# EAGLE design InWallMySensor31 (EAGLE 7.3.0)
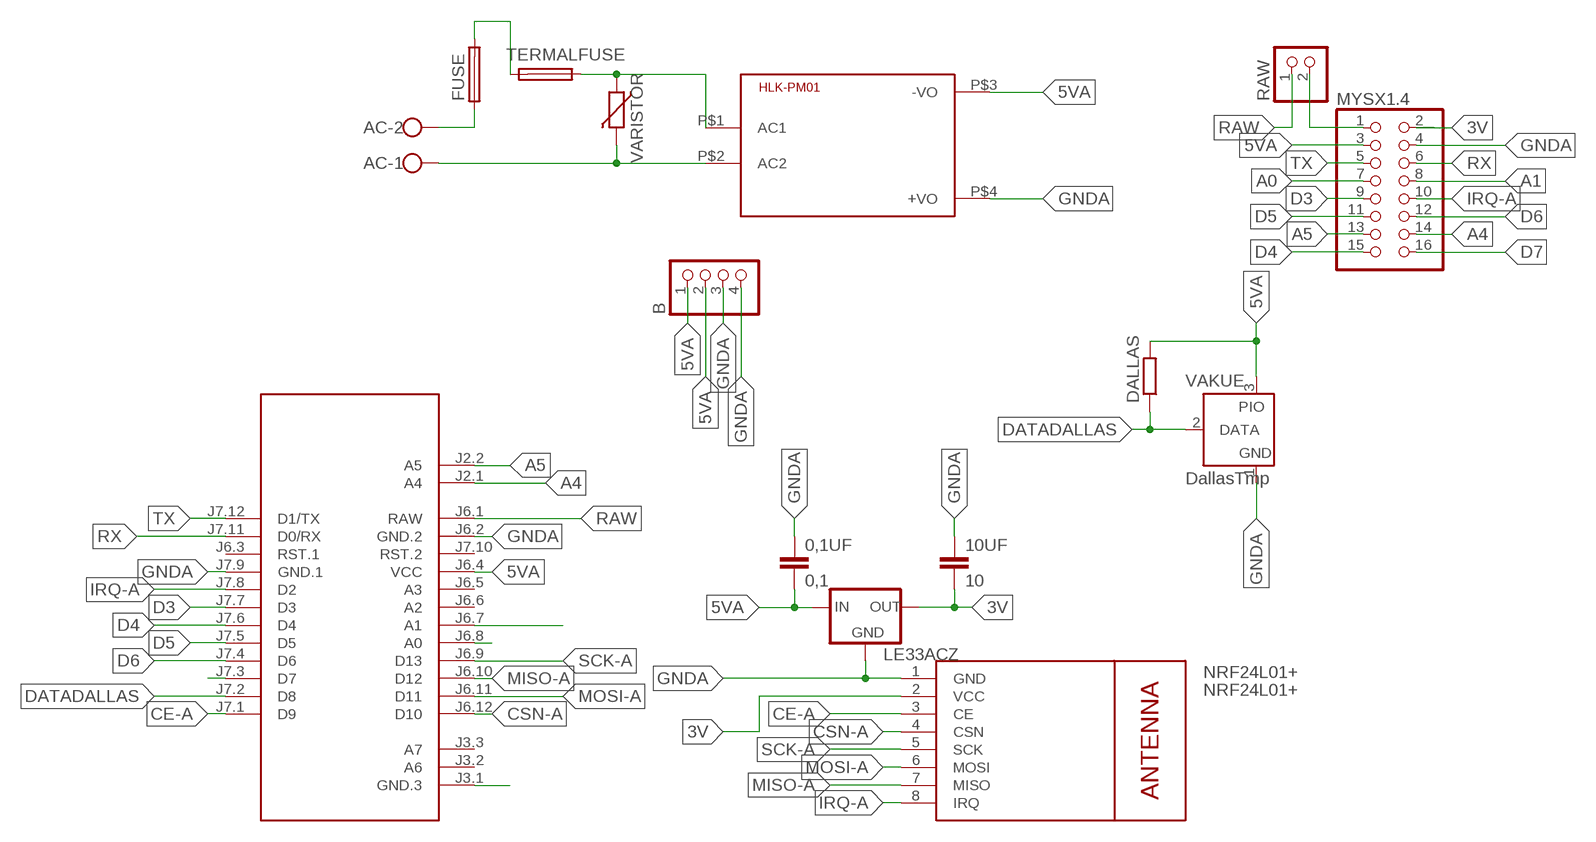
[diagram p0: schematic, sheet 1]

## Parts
0,1UF  0,1  C5/2.5  [C5B2.5]
10UF  10  C5/2.5  [C5B2.5]
AC  W237-102  [W237-102]
B  PINHD-1X04_2.54-S  [1X04-S]
DALLAS  R-EU_0204/5  [0204/5]
FUSE  FUSETE5  [TE5]
HLK-PM01  HKLPM01  [HKLPM01]
LE33ACZ  78LXX  [78LXX]
M1  ARDUINO-PRO-MINI-3.3V#NP  [ARDUINO-PRO-MINI#NP]
MYSX1.4  PINHD-2X08_2.54  [2X08]
NRF24L01+  NRF24L01+  WIRELESS-NRF24L01  [WIRELESS-NRF24L01]
RAW  PINHD-1X02_2.54-S  [1X02-S]
TERMALFUSE  FUSETE5  [TE5]
VAKUE  DallasTmp  DS2405  [TO92-]
VARISTOR  VARISTOR-7,5  [R-7,5]

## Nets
3V: 10UF.2 LE33ACZ.OUT MYSX1.4.2 NRF24L01+.2(VCC)
5VA: 0,1UF.2 B.1 B.2 DALLAS.2 HLK-PM01.P$3(-VO) LE33ACZ.IN M1.J6.4(VCC) MYSX1.4.3 VAKUE.3(PIO)
A0: M1.J6.8(A0) MYSX1.4.7
A1: M1.J6.7(A1) MYSX1.4.8
A4: M1.J2.1(A4) MYSX1.4.14
A5: M1.J2.2(A5) MYSX1.4.13
ACGND: AC.1 HLK-PM01.P$2(AC2) VARISTOR.2
CE-A: M1.J7.1(D9) NRF24L01+.3(CE)
CSN-A: M1.J6.12(D10) NRF24L01+.4(CSN)
D3: M1.J7.7(D3) MYSX1.4.9
D4: M1.J7.6(D4) MYSX1.4.15
D5: M1.J7.5(D5) MYSX1.4.11
D6: M1.J7.4(D6) MYSX1.4.12
D7: M1.J7.3(D7) MYSX1.4.16
DATADALLAS: DALLAS.1 M1.J7.2(D8) VAKUE.2(DATA)
GNDA: 0,1UF.1 10UF.1 B.3 B.4 HLK-PM01.P$4(+VO) LE33ACZ.GND M1.J6.2(GND.2) M1.J7.9(GND.1) MYSX1.4.4 NRF24L01+.1(GND) VAKUE.1(GND)
IRQ-A: M1.J7.8(D2) MYSX1.4.10 NRF24L01+.8(IRQ)
MISO-A: M1.J6.10(D12) NRF24L01+.7(MISO)
MOSI-A: M1.J6.11(D11) NRF24L01+.6(MOSI)
N$1: FUSE.2 TERMALFUSE.2
N$4: AC.2 FUSE.1
N$5: M1.J3.1(GND.3)
N$6: MYSX1.4.1 RAW.2
N$7: HLK-PM01.P$1(AC1) TERMALFUSE.1 VARISTOR.1
RAW: M1.J6.1(RAW) RAW.1
RX: M1.J7.11(D0/RX) MYSX1.4.6
SCK-A: M1.J6.9(D13) NRF24L01+.5(SCK)
TX: M1.J7.12(D1/TX) MYSX1.4.5
Unconnected: M1.J3.2(A6) M1.J3.3(A7) M1.J6.3(RST.1) M1.J6.5(A3) M1.J6.6(A2) M1.J7.10(RST.2)

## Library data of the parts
0,1UF 10UF = capacitor-wima:C: CAPACITOR
AC = con-wago-500:W237-102: WAGO SCREW CLAMP; MPN: 237-102; OC_FARNELL: unknown; OC_NEWARK: 70K9898
B = pinhead-2:PINHD-1X04: PIN HEADER
DALLAS = resistor:R-EU_: RESISTOR, European symbol
FUSE TERMALFUSE = fuse:FUSE: Fuse; OC_FARNELL: unknown; OC_NEWARK: unknown
HLK-PM01 = HKLPM01:HKLPM01
LE33ACZ = v-reg:78LXX: VOLTAGE REGULATOR
M1 = diy-modules:ARDUINO-PRO-MINI-*#NP: Arduino Pro Mini without programming pads
MYSX1.4 = pinhead-2:PINHD-2X08: PIN HEADER
NRF24L01+ = diy-modules:WIRELESS-NRF24L01: 2.4 GHz Wireless Module based on NRF24L01 chip
RAW = pinhead-2:PINHD-1X02: PIN HEADER
VAKUE = maxim:DS2405: Addressable Switch DALLAS Semiconductor; MF: DALLAS SEMICONDUCTOR; MPN: DS2405; OC_FARNELL: 1188025; OC_NEWARK: 06F4645
VARISTOR = varistor:VARISTOR: VARISTOR

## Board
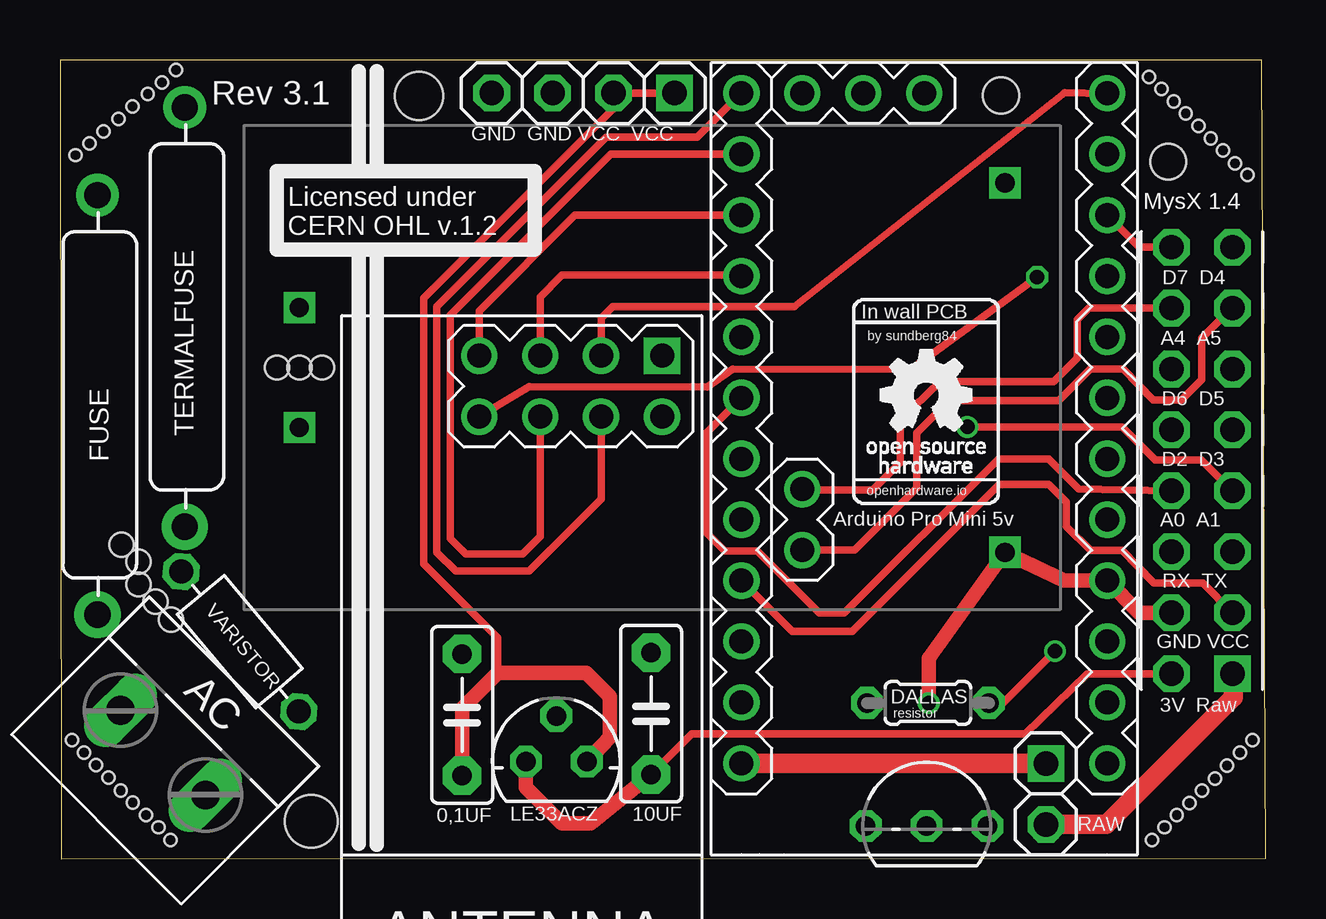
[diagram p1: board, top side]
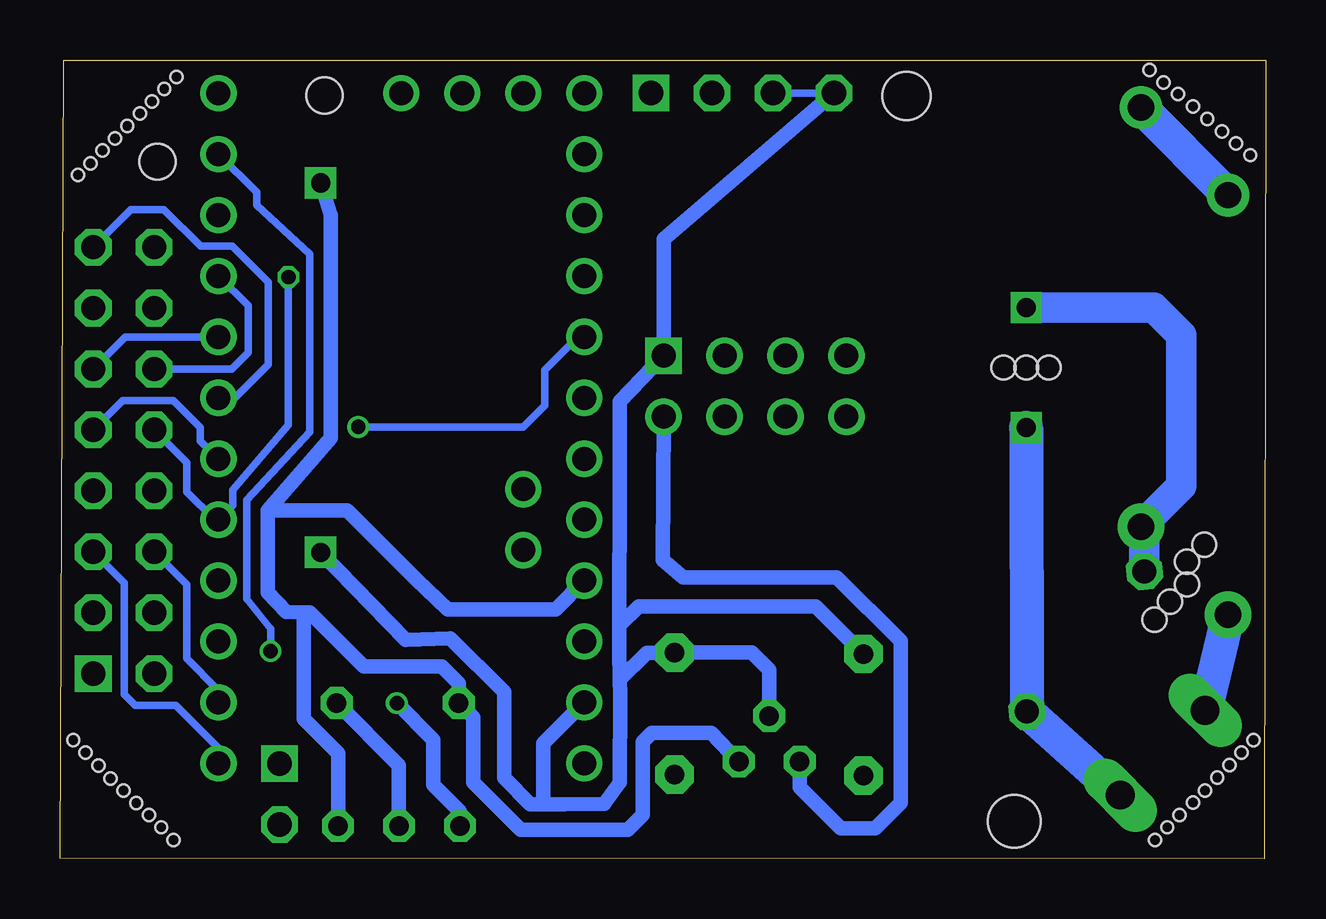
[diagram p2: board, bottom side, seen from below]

Size 50.23 x 33.31 mm. Coordinates in mm from the lower left corner, seen from the top.
Outline: 0.05,0 50.23,0.03 50.08,33.31 0,33.31 0.05,0
Copper layers (1*16): Top 0.035mm / dielectric 1.5mm / Bottom 0.035mm
Design rules "ITead_rule": minimum track width 6mil, minimum drill 12mil, track to track 6mil, track to pad 6mil, pad to pad 6mil, via to via 6mil, smd to smd 0mil, copper to edge 10mil, drill to drill 10mil, minimum pad ring 10mil, minimum via ring 6mil, stop-mask expansion 2mil, vias tented up to drill 100mil, thermal gap 10mil
Holes 2 mm at 14.96,31.81
Holes 2.2 mm at 10.47,1.56
Holes 1.5 mm at 39.2,31.83 46.18,29.07
Holes 0.5 mm at 45.38,32.61 46.41,31.58 47.43,30.56 48.46,29.53 49.48,28.51 45.51,0.78 46.53,1.83 47.58,2.86 48.63,3.88 49.68,4.96 4.61,0.78 3.58,1.83 2.53,2.86 1.51,3.91 0.51,4.96 4.83,32.88 3.66,31.88 2.43,30.86 1.23,29.83 4.1,1.32 3.03,2.36 2.02,3.4 1,4.44 0.64,29.34 1.81,30.33 3.03,31.37 4.25,32.36 45.89,32.1 46.91,31.08 47.95,30.04 48.96,29 46.01,1.32 47.06,2.33 48.12,3.35 49.16,4.44
Holes 1 mm at 3.27,12.38 3.27,11.44 3.98,10.73 9.97,20.48 9.03,20.48 10.91,20.48 2.56,13.09 4.63,9.98

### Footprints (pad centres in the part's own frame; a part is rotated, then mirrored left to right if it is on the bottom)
C5B2.5 = drill 0.813 pad 1.6 octagon: 1 -2.54,0; 2 2.54,0
W237-102 = drill 1.194 long: 1 -2.5,-1.27; 2 2.5,-1.27
1X04-S = drill 1.016 square: 1 -3.81,0 | drill 1.016 octagon: 2 -1.27,0; 3 1.27,0; 4 3.81,0
0204/5 = drill 0.813 octagon: 1 -2.54,0; 2 2.54,0
TE5 = drill 1.1 pad 1.93: 1 -5.632,0 | drill 1.1 pad 1.778: 2 11.852,0
HKLPM01 = drill 0.8 square: P$1 -14.7,2.5; P$2 -14.7,-2.5; P$3 14.7,7.7; P$4 14.7,-7.7
78LXX = drill 0.813 octagon: GND 0,1.905; IN 1.27,0; OUT -1.27,0
ARDUINO-PRO-MINI#NP = drill 1: J2.1 -1.27,5.08; J2.2 -3.81,5.08; J3.1 15.24,0; J3.2 15.24,2.54; J3.3 15.24,5.08; J6.1 -12.7,7.62; J6.2 -10.16,7.62; J6.3 -7.62,7.62; J6.4 -5.08,7.62; J6.5 -2.54,7.62; J6.6 0,7.62; J6.7 2.54,7.62; J6.8 5.08,7.62; J6.9 7.62,7.62; J6.10 10.16,7.62; J6.11 12.7,7.62; J6.12 15.24,7.62; J7.1 15.24,-7.62; J7.2 12.7,-7.62; J7.3 10.16,-7.62; J7.4 7.62,-7.62; J7.5 5.08,-7.62; J7.6 2.54,-7.62; J7.7 0,-7.62; J7.8 -2.54,-7.62; J7.9 -5.08,-7.62; J7.10 -7.62,-7.62; J7.11 -10.16,-7.62; J7.12 -12.7,-7.62
2X08 = drill 1.016 square: 1 -8.89,-1.27 | drill 1.016 octagon: 2 -8.89,1.27; 3 -6.35,-1.27; 4 -6.35,1.27; 5 -3.81,-1.27; 6 -3.81,1.27; 7 -1.27,-1.27; 8 -1.27,1.27; 9 1.27,-1.27; 10 1.27,1.27; 11 3.81,-1.27; 12 3.81,1.27; 13 6.35,-1.27; 14 6.35,1.27; 15 8.89,-1.27; 16 8.89,1.27
WIRELESS-NRF24L01 = drill 1 square: 1 -12.7,6.35 | drill 1: 2 -10.16,6.35; 3 -12.7,3.81; 4 -10.16,3.81; 5 -12.7,1.27; 6 -10.16,1.27; 7 -12.7,-1.27; 8 -10.16,-1.27
1X02-S = drill 1.016 square: 1 -1.27,0 | drill 1.016 octagon: 2 1.27,0
TO92- = drill 0.813 octagon: 1 -2.54,0; 2 0,0; 3 2.54,0
R-7,5 = drill 1 octagon: 1 -3.81,0; 2 3.81,0

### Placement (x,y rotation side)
0,1UF  16.76,6.01 270 top
10UF  24.63,6.06 270 top
AC  3.39,3.53 135 top
B  21.8,31.93 180 top
DALLAS  36.16,6.5 180 top
FUSE  1.56,15.82 90 top
HLK-PM01  24.67,20.48 0 top
LE33ACZ  20.68,4.06 0 top
M1  36.01,16.68 90 top
MYSX1.4  47.58,16.61 90 top
NRF24L01+  18.73,8.28 270 top
RAW  41.08,2.71 270 top
TERMALFUSE  5.2,19.48 90 top
VAKUE  36.11,1.37 0 top
VARISTOR  7.5,9.06 310 top

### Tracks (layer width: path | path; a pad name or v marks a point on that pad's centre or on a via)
3V
  Top 0.305: MYSX1.4.2 42.8,7.72 40.21,5.22 26.33,5.22 10UF.2
  Top 0.61: 10UF.2 22.12,1.48 20.91,1.48 19.41,2.98 LE33ACZ.OUT
  Bottom 0.61: NRF24L01+.2 25.11,12.47 24.27,11.74 17.86,11.74 15.21,9.08 15.21,2.33 16.26,1.28 17.71,1.28 19.41,2.98 LE33ACZ.OUT
5VA
  Top 0.305: 18.23,7.76 18.23,9.21 15.16,12.29 15.16,23.38 23.07,31.3 B.2 B.1 | MYSX1.4.3 47.6,11.51 45.58,11.51 44.26,12.86 42.96,12.86 41.93,13.86 41.93,14.88 41.2,15.61 39.13,15.61 33.01,9.48 30.51,9.48 M1.J6.4
  Top 0.61: 0,1UF.2 16.76,6.28 18.23,7.76 21.93,7.76 22.91,6.78 22.91,5.06 LE33ACZ.IN
  Bottom 0.61: 41.57,14.53 38.27,14.53 35.4,11.66 34.07,10.41 29.59,10.41 M1.J6.4 | 41.57,14.53 41.57,13.23 41.57,11.1 40.8,10.31 40.26,10.28 | LE33ACZ.IN 23.1,5.25 25.58,5.25 25.96,4.88 25.96,1.83 26.58,1.21 31.04,1.21 33.02,3.2 33.02,5.91 DALLAS.2 33.62,7.32 34.32,8.02 37.57,8.02 39.83,10.28 40.26,10.28 | VAKUE.3 38.65,4.4 40.09,5.84 40.09,10.1 40.26,10.28 | HLK-PM01.P$3 38.95,26.83 38.95,17.55 41.57,14.53
A0  (via drill 0.6)
  Top 0.305: MYSX1.4.7 47.56,16.63 45.63,16.63 44.26,18.01 v37.81,18.01
  Bottom 0.305: M1.J6.8 28.65,21.76 30.03,20.38 30.03,18.91 30.93,18.01 v37.81,18.01
A1
  Top 0.305: MYSX1.4.8 42.45,15.42 41.21,16.68 39.11,16.68 32.68,10.26 31.63,10.26 29.06,12.83 27.71,12.83 26.91,13.63 26.91,17.74 M1.J6.7
A4
  Top 0.305: MYSX1.4.14 42.86,22.96 42.38,22.48 42.38,20.88 41.41,19.91 36.68,19.91 35.01,18.29 35.01,16.53 33.86,15.38 30.96,15.38 M1.J2.1
A5
  Top 0.305: M1.J2.2 33.12,12.87 35.71,15.46 35.71,17.76 37.06,19.11 41.61,19.11 42.93,20.43 44.3,20.43 45.56,19.12 46.72,19.12 47.58,19.98 47.58,21.71 48.83,22.96 MYSX1.4.13
ACGND
  Bottom 1.422: HLK-PM01.P$2 VARISTOR.2 AC.1
CE-A
  Top 0.305: NRF24L01+.3 22.54,22.55 23.03,23.03 30.59,23.03 41.87,31.93 43.62,31.91 M1.J7.1
CSN-A
  Top 0.305: M1.J6.12 26.55,30.08 22.76,30.08 15.71,23.03 15.71,12.78 16.48,12.01 19.55,12.01 22.54,15 NRF24L01+.4
D3
  Bottom 0.305: MYSX1.4.9 47.62,19.11 45.51,19.11 44.38,17.98 44.38,17.43 M1.J7.7
D4
  Bottom 0.305: M1.J7.6 42.95,19.22 41.56,20.62 41.56,24.05 43.06,25.55 44.38,25.55 45.9,27.07 47.28,27.07 MYSX1.4.15
D5
  Bottom 0.305: MYSX1.4.11 47.51,21.76 M1.J7.5
D6
  Bottom 0.305: MYSX1.4.12 43.08,20.42 42.4,21.1 42.4,23.07 M1.J7.4
D7
  Top 0.305: MYSX1.4.16 44.97,25.5 M1.J7.3
DATADALLAS  (via drill 0.6)
  Top 0.305: DALLAS.1 39.3,6.5 v41.46,8.66
  Bottom 0.305: v41.46,8.66 41.46,9.59 42.45,10.84 42.45,14.96 39.83,17.8 39.83,25.22 42.04,27.25 42.04,27.79 M1.J7.2
  Bottom 0.61: VAKUE.2 36.11,3.91 DALLAS.1
GNDA  (via drill 0.6)
  Top 0.61: MYSX1.4.4 44.97,10.26 M1.J7.9 41.83,11.6 HLK-PM01.P$4 36.2,8.36 v36.2,6.5
  Bottom 0.305: B.4 B.3
  Bottom 0.61: 26.92,9.73 26.91,15.8 26.91,19.07 NRF24L01+.1 25.08,25.83 B.4 | 26.92,9.73 26.93,8.88 26.93,8.61 26.91,7.48 | 26.91,7.48 26.9,6.83 26.91,3.2 27.55,2.29 29.22,2.28 30.11,2.28 | M1.J6.2 30.11,4.81 30.11,2.28 | LE33ACZ.GND 20.68,7.88 21.41,8.61 24.09,8.61 10UF.1 25.79,8.6 26.91,7.48 | 30.11,2.28 30.64,2.28 31.73,3.37 31.73,6.95 33.96,9.19 35.83,9.14 HLK-PM01.P$4 | VAKUE.1 33.57,1.99 34.68,3.09 34.68,4.97 v36.2,6.5 | 26.92,9.73 26.12,10.53 18.74,10.53 0,1UF.1
IRQ-A  (via drill 0.6)
  Top 0.305: NRF24L01+.8 19.55,19.69 26.98,19.67 28.02,20.41 35.46,20.39 v40.72,24.26
  Bottom 0.305: MYSX1.4.10 44.96,16.53 44.96,15.31 43.79,14.14 M1.J7.8 43.03,14.74 43.03,15.39 40.72,18.08 v40.72,24.26
MISO-A
  Top 0.305: NRF24L01+.7 17.46,22.84 21.46,26.83 28.38,26.83 M1.J6.10
MOSI-A
  Top 0.305: M1.J6.11 22.96,29.38 16.26,22.68 16.26,13.36 16.91,12.71 19.27,12.71 20,13.44 NRF24L01+.6
N$1
  Bottom 1.422: FUSE.2 TERMALFUSE.2
N$4
  Bottom 1.422: FUSE.1 AC.2
N$6
  Top 0.813: MYSX1.4.1 48.88,7.69 48.88,6.73 43.59,1.44 RAW.2
N$7
  Bottom 1.27: HLK-PM01.P$1 4.65,22.98 3.51,21.84 3.51,15.54 TERMALFUSE.1 5.05,13.7 VARISTOR.1
RAW
  Top 0.813: M1.J6.1 RAW.1
RX
  Bottom 0.305: MYSX1.4.6 44.96,11.45 44.96,8.36 43.63,7.03 M1.J7.11
SCK-A
  Top 0.305: NRF24L01+.5 20,23.43 20.91,24.33 28.36,24.33 M1.J6.9
TX
  Bottom 0.305: MYSX1.4.5 47.56,11.51 47.56,6.86 47.11,6.41 45.41,6.41 43.63,4.63 M1.J7.12

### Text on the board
tPlace: GND GND VCC VCC | Licensed under / CERN OHL v.1.2 | D7 D4 | In wall PCB | by sundberg84 | A4 A5 | D6 D5 | D2 D3 | openhardware.io | A0 A1 | RX TX | GND VCC | 3V Raw
tNames: Rev 3.1 | MysX 1.4 | Arduino Pro Mini 5v | resistor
